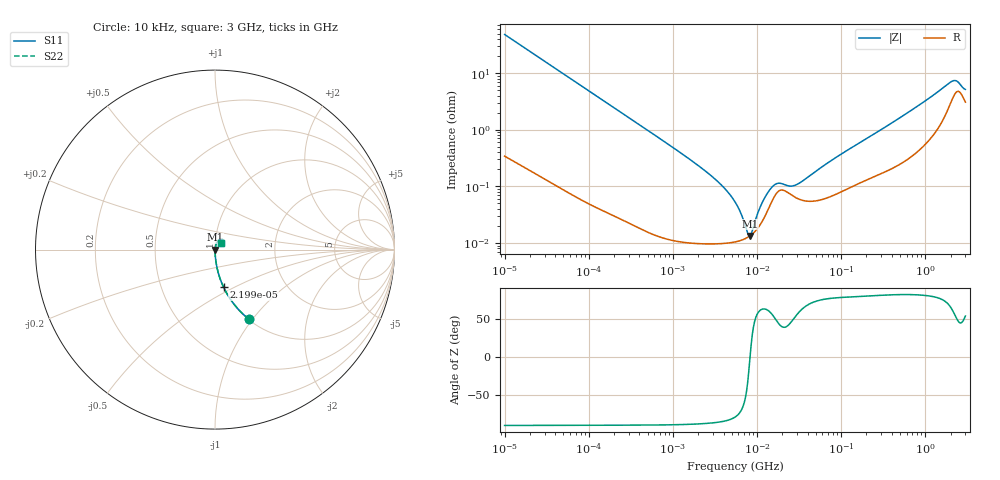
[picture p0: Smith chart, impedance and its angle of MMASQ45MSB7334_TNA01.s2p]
! MMASQ45MSB7334_TNA01  S-PARAMETER MODEL  ( Standard Model )
! Model Generated by TAIYO YUDEN Corporation (http://www.ty-top.com)
! Version 1.0
! TAIYO YUDEN Control No. 220601
! Copyright(c) 2013 TAIYO YUDEN CO.,LTD. All Rights Reserved.
! Product Description (link to TY-COMPAS)
! https://ds.yuden.co.jp/TYCOMPAS/or/detail?pn=MMASQ45MSB7334KTNA01&u=M
! Products Name : Multilayer Ceramic Capacitors
! Characteristics :
!  Capacitance : 0.33 [uF] , Rated Voltage : 250 [V] , TCC : X7R
!  Case Size : 4.5 x 3.2 / 0.177 x 0.126 [mm/inch] , Thickness : 2.5 / 0.098 [mm/inch]
!  (Conditions: Temperature = 25 [degC] , DC Bias Voltage = 0 [V])
! External Node Assignments :
!  1  o---| |---o  2
! GND o---------o GND
! Frequency Range : 10kHz  -  3GHz  [ 401 STEP ]
# MHZ S RI R 50
! Freq[MHz].  S11 Real  S11 Imag  S21 Real  S21 Imag  S12 Real  S12 Imag  S22 Real  S22 Imag
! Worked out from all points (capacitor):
!   401 points, 10 kHz to 3 GHz, reference 50 ohm
!   read as one part in series: C = 330 nF near 10.65 kHz
!   lowest |Z| = 13.4 mohm at 8.252 MHz (marker M1)
!   series resonance near 8.268 MHz, so ESL is about 1.1 nH
!   S11 on the Smith chart (normalised r, x): 10 kHz: 1.01, -0.96; 22 kHz: 1.00, -0.44; 3 GHz: 1.06, +0.08
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0.01  0.1897 -0.3885  0.8103 0.3885  0.8103 0.3885  0.1897 -0.3885
0.021995  0.0475 -0.2087  0.9525 0.2087  0.9525 0.2087  0.0475 -0.2087
0.082683  0.00401 -0.0585  0.996 0.0585  0.996 0.0585  0.00401 -0.0585
0.683653  0.00018 -0.00715  0.9998 0.00715  0.9998 0.00715  0.00018 -0.00715
2.824956  9.86e-05 -0.00156  0.9999 0.00156  0.9999 0.00156  9.86e-05 -0.00156
4.124064  9.92e-05 -0.000915  0.9999 0.000915  0.9999 0.000915  9.92e-05 -0.000915
5.477226  0.000104 -0.000522  0.9999 0.000522  0.9999 0.000522  0.000104 -0.000522
6.41246  0.000111 -0.000321  0.9999 0.000321  0.9999 0.000321  0.000111 -0.000321
7.747855  0.000126 -8.28e-05  0.9999 8.28e-05  0.9999 8.28e-05  0.000126 -8.28e-05
8.252149  0.000133 -2.42e-06  0.9999 2.42e-06  0.9999 2.42e-06  0.000133 -2.42e-06
8.789267  0.000144 7.93e-05  0.9999 -7.93e-05  0.9999 -7.93e-05  0.000144 7.93e-05
10.29003  0.000185 0.000293  0.9998 -0.000293  0.9998 -0.000293  0.000185 0.000293
11.67315  0.000248 0.000475  0.9998 -0.000475  0.9998 -0.000475  0.000248 0.000475
13.66633  0.000399 0.000698  0.9996 -0.000698  0.9996 -0.000698  0.000399 0.000698
15.50326  0.000596 0.000816  0.9994 -0.000816  0.9994 -0.000816  0.000596 0.000816
18.15044  0.000827 0.000778  0.9992 -0.000778  0.9992 -0.000778  0.000827 0.000778
28.22191  0.000644 0.000819  0.9994 -0.000819  0.9994 -0.000819  0.000644 0.000819
45.28751  0.000547 0.00156  0.9995 -0.00156  0.9995 -0.00156  0.000547 0.00156
374.4521  0.0021 0.0122  0.9979 -0.0122  0.9979 -0.0122  0.0021 0.0122
2054.98  0.035 0.0592  0.965 -0.0592  0.965 -0.0592  0.035 0.0592
2331.196  0.0467 0.052  0.9533 -0.052  0.9533 -0.052  0.0467 0.052
3000  0.0314 0.0388  0.9686 -0.0388  0.9686 -0.0388  0.0314 0.0388
